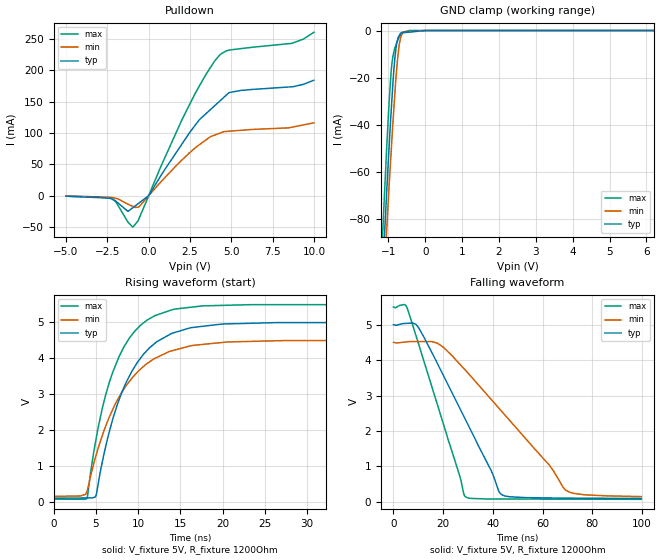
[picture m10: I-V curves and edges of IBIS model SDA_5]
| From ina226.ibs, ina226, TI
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[Model]   SDA_5
Model_type   I/O_open_drain
Polarity   Non-Inverting
Enable   Active-Low
Vinl = 1.5
Vinh = 3.5
Vmeas = 2.5
Vref = 2.5
Cref = 2pF
Rref = 1200
|   typ   min   max
|   (nom PVT)   (Fast PVT)   (slow PVT)
|   ON state : BUFFER OUTPUT TURNED HIGH
C_comp   1.175E-12   9.640E-13   1.381E-12
|   OFF state: BUFFER OUTPUT TURNED LOW
|C_comp   8.711E-13   8.711E-13   1.009E-12
| Where   nom PVT is  Nominal Process, 3.3V, 25C
|   Fast PVT is Strong Process, 3.6V, -40C
|   Slow PVT is Weak Process, 3.0V, 85C
|C_comp - from L-C Tank method, L = 1nH, peak frequency
[Model Spec]
| variable   typ   min   max
Vinl   1.5   1.35   1.65
Vinh   3.5   3.15   3.85
|Vinl = 0.3 x V+, Vinh = 0.7 x V+
[Voltage Range]   5   4.5   5.5
|Ambient Temperature Range   27   85   -40
[Temperature Range]   30   88   -40
[Pullup Reference]   5   4.5   5.5
[Pulldown Reference]   0   0   0
[Power Clamp Reference]   5   4.5   5.5
[GND Clamp Reference]   0   0   0
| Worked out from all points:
|   slope of the pulldown table from 0 to 0.75 V, typ, clamps not added: 23.2 ohm
|   GND clamp passes 1 mA (typ) near -0.65 V on its own axis
|   falling waveform, V_fixture 5V, R_fixture 1200Ohm: 20-80 % time 21ns typ, 32.8ns min, 14.4ns max; typ from 5 V to 0.097 V
|   rising waveform, V_fixture 5V, R_fixture 1200Ohm: 20-80 % time 4.6ns typ, 5.28ns min, 3.97ns max; typ from 0.097 V to 5 V
[Pulldown]
|   Voltage   I(typ)   I(min)   I(max)
-5V       -741uA     -571uA     -728.2uA
-2.197V   -5.474mA   -2.77mA    -4.853mA
-1.253V   -24.89mA   -13.44mA   -41.92mA
-957.8mV  -19.03mA   -16.89mA   -50.02mA
-600.9mV  -11.93mA   -17.92mA   -37.54mA
532.3uV   23.43uA    16.25uA    26.47uA
2.625V    105.7mA    71.81mA    153.2mA
3.49V     131.2mA    89.32mA    194.1mA
4.326V    151.3mA    99.82mA    224.9mA
4.863V    164.2mA    102.7mA    231.9mA
8.643V    173.4mA    109mA      242.5mA
9.985V    183.9mA    116mA      260.1mA
[GND Clamp]
|   Voltage   I(typ)   I(min)   I(max)
-5V       -1.381A    -1.301A    -1.543A
-1.238V   -127.5mA   -139.2mA   -115.5mA
-1.125V   -92.84mA   -107.1mA   -75.92mA
-1.043V   -67.65mA   -83.79mA   -48.79mA
-976.5mV  -48.25mA   -64.87mA   -29.21mA
-925.2mV  -34.28mA   -51.46mA   -17.45mA
-883.5mV  -23.87mA   -40.6mA    -11.48mA
-824.9mV  -11.71mA   -26.81mA   -7.472mA
-777mV    -5.587mA   -16.72mA   -5.429mA
-712.9mV  -2.278mA   -6.735mA   -3.011mA
-618.2mV  -951.4uA   -1.13mA    -715.7uA
9.985V    0A         0A         0A
[POWER Clamp]
|   SCR cell for ESD function. Effects occurr above VDD x 2
|   Voltage   I(typ)   I(min)   I(max)
-5V       0A         0A         0A
0V        0A         0A         0A
10V       0A         0A         0A
[Ramp]
R_load = 1200
|   typ   min   max
dV/dt_r   2.94187/4.58941e-009   2.61084/5.27516e-009   3.25746/3.96421e-009
dV/dt_f   2.94185/2.10128e-008   2.61066/3.28221e-008   3.25745/1.44365e-008
[Falling Waveform]
V_fixture = 5V
V_fixture_min = 4.5V
V_fixture_max = 5.5V
R_fixture = 1200Ohm
C_fixture = 0F
|   Time   V(typ)   V(min)   V(max)
0s        5V         4.5V       5.5V
4.38ns    5.036V     4.508V     5.571V
5.517ns   5.04V      4.517V     5.472V
10.22ns   4.907V     4.525V     4.434V
17.66ns   3.91V      4.481V     2.75V
29.02ns   2.315V     3.71V      141.7mV
43.49ns   205.4mV    2.558V     79.65mV
62.78ns   109.7mV    1.029V     76.65mV
69.74ns   103.8mV    309.1mV    75.57mV
99.71ns   96.92mV    148.9mV    70.9mV
[Rising Waveform]
V_fixture = 5V
V_fixture_min = 4.5V
V_fixture_max = 5.5V
R_fixture = 1200Ohm
C_fixture = 0F
|   Time   V(typ)   V(min)   V(max)
0s        96.88mV    148.6mV    70.9mV
3.957ns   103.8mV    284.1mV    89.47mV
4.969ns   137.2mV    1.244V     1.665V
5.738ns   1.069V     1.82V      2.571V
6.625ns   1.972V     2.376V     3.35V
8.612ns   3.34V      3.244V     4.427V
11.34ns   4.287V     3.897V     5.102V
14.05ns   4.699V     4.212V     5.355V
26.31ns   4.994V     4.488V     5.496V
99.71ns   5V         4.5V       5.5V
